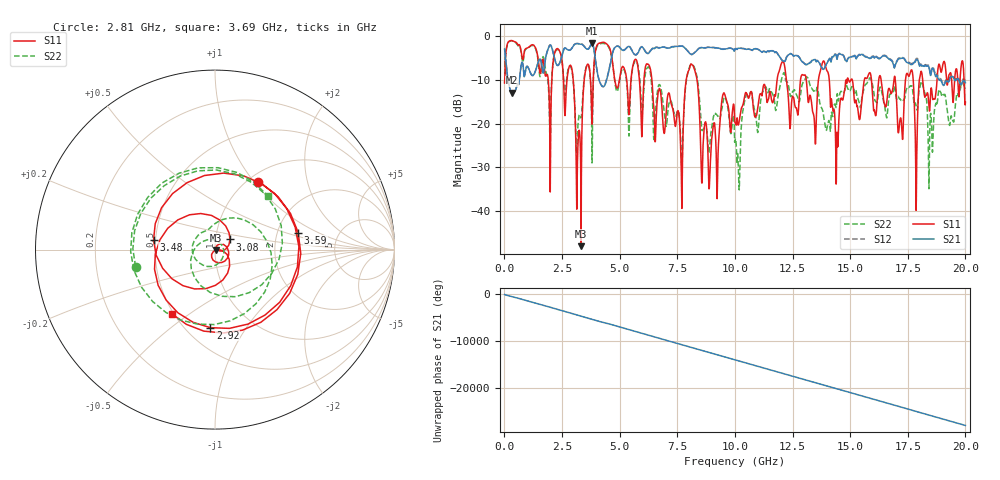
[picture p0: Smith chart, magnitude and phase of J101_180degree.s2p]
!Keysight Technologies,N5222A,MY51421036,A.10.65.16
!Date: Friday, March 31, 2023 14:50:38
!Correction: S11(Full 2 Port(1,2))
!S21(Full 2 Port(1,2))
!S12(Full 2 Port(1,2))
!S22(Full 2 Port(1,2))
!S2P File: Measurements: S11, S21, S12, S22:
# Hz S  dB  R 50
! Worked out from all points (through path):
!   2000 points, 10 MHz to 20 GHz, reference 50 ohm
!   highest |S21| = -1.59 dB at 3.8 GHz (marker M1); lowest = -12.9 dB at 340 MHz (marker M2)
!   group delay of S21, straight-line fit = 3.9 ns
!   lowest |S11| = -48.0 dB at 3.33 GHz (marker M3), VSWR 1.01, Z = 50.3 - j0.242 ohm
!   |S11| at or under -10 dB: 6.4 GHz to 7.887 GHz (1.487 GHz wide, 20.8 % of centre); 8.36 GHz to 11.83 GHz (3.47 GHz wide, 34.4 % of centre); 14.1 GHz to 14.82 GHz (721.7 MHz wide, 4.99 % of centre)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
!   |S22| runs from -35.1 to -1.0 dB; largest |S21 - S12| = 0.023
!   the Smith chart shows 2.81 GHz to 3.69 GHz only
!   S11 on the Smith chart (normalised r, x): 2.81 GHz: 1.11, +1.05; 2.92 GHz: 0.65, -0.70; 3.08 GHz: 1.17, +0.13; 3.48 GHz: 0.49, +0.06; 3.59 GHz: 2.62, +0.64; 3.69 GHz: 0.49, -0.43
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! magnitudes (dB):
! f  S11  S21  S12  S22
! 10 MHz  -10.7  -2.9  -2.9  -10.6
! 340 MHz  -1.0  -12.9  -12.8  -1.0
! 1.95 GHz  -15.0  -2.2  -2.1  -16.7
! 2.81 GHz  -7.0  -3.2  -3.1  -6.9
! 2.92 GHz  -7.2  -2.8  -2.7  -7.6
! 3.08 GHz  -19.9  -1.7  -1.7  -19.5
! 3.33 GHz  -48.0  -1.8  -1.7  -18.6
! 3.35 GHz  -26.6  -1.8  -1.7  -17.7
! 3.48 GHz  -9.2  -2.4  -2.3  -8.8
! 3.59 GHz  -6.5  -2.9  -2.8  -6.6
! 3.69 GHz  -7.3  -2.6  -2.5  -7.5
! 3.8 GHz  -20.1  -1.6  -1.5  -29.0
! 4.24 GHz  -1.4  -11.4  -11.4  -1.6
! 6.68 GHz  -12.7  -2.7  -2.6  -11.3
! 7.68 GHz  -32.7  -2.2  -2.2  -29.1
! 8.17 GHz  -6.6  -4.1  -4.0  -6.4
! 8.9 GHz  -33.3  -2.5  -2.5  -25.3
! 10.01 GHz  -19.8  -2.9  -2.8  -23.9
! 12.06 GHz  -5.8  -5.5  -5.5  -9.1
! 13.34 GHz  -15.9  -5.6  -5.5  -11.9
! 16.67 GHz  -11.9  -5.1  -5.0  -14.5
! 20 GHz  -15.1  -10.6  -10.2  -11.8
